{attribute 'qualified_only'}
VAR_GLOBAL
//######################## EL1809 ########################
	I_bTerm1_Var1 AT%I* : BOOL;		// Kitchen Light1
	I_bTerm1_Var2 AT%I* :  BOOL;	// Kitchen Light2
	I_bTerm1_Var3 AT%I* : BOOL;		// Kitchen Light3
	I_bTerm1_Var4 AT%I* : BOOL;		// Kitchen Blind Up
	I_bTerm1_Var5 AT%I* : BOOL;		// Kitchen Blind Down
	I_bTerm1_Var6 AT%I* : BOOL;
	I_bTerm1_Var7 AT%I* : BOOL;		// Corridor Light1
	I_bTerm1_Var8 AT%I* : BOOL;		// Corridor Light2
	I_bTerm1_Var9 AT%I* : BOOL;
	I_bTerm1_Var10 AT%I*:  BOOL;	// Livingroom Light1
	I_bTerm1_Var11 AT%I*:  BOOL;	// Livingroom Light2
	I_bTerm1_Var12 AT%I* : BOOL;	// Livingroom Light3
	I_bTerm1_Var13 AT%I* : BOOL;	// Livingroom Blind1 Up
	I_bTerm1_Var14 AT%I* : BOOL;	// Livingroom Blind1 Down
	I_bTerm1_Var15 AT%I* : BOOL;	// Livingroom Blind2 Up
	I_bTerm1_Var16 AT%I* : BOOL;	// Livingroom Blind2 Down
	
//######################## EL1809 ########################
	I_bTerm2_Var1 AT%I* : BOOL;		// Diningroom Light1
	I_bTerm2_Var2 AT%I* :  BOOL;	// Diningroom Light2
	I_bTerm2_Var3 AT%I* : BOOL;		// Diningroom Light3
	I_bTerm2_Var4 AT%I* : BOOL;		// Diningroom Blind1 Up
	I_bTerm2_Var5 AT%I* : BOOL;		// Diningroom Blind1 Down
	I_bTerm2_Var6 AT%I* : BOOL;		// Diningroom Blind2 Up
	I_bTerm2_Var7 AT%I* : BOOL;		// Diningroom Blind2 Down
	I_bTerm2_Var8 AT%I* : BOOL;
	I_bTerm2_Var9 AT%I* : BOOL;		// Bedroom Light1
	I_bTerm2_Var10 AT%I*:  BOOL;	// Bedroom Light2
	I_bTerm2_Var11 AT%I*:  BOOL;	// Bedroom Blind Up
	I_bTerm2_Var12 AT%I* : BOOL;	// Bedroom Blind Down
	I_bTerm2_Var13 AT%I* : BOOL;
	I_bTerm2_Var14 AT%I* : BOOL;	// Bath Light
	I_bTerm2_Var15 AT%I* : BOOL;	// Bath Blind Up
	I_bTerm2_Var16 AT%I* : BOOL;	// Bath Blind Down
	
//######################## EL2809 ########################
	Q_bTerm3_Var1 AT%Q* : BOOL;		// Kitchen Light1 ON
	Q_bTerm3_Var2 AT%Q* :  BOOL;	// Kitchen Light2 ON
	Q_bTerm3_Var3 AT%Q* : BOOL;		// Kitchen Light3 ON
	Q_bTerm3_Var4 AT%Q* : BOOL;		
	Q_bTerm3_Var5 AT%Q* : BOOL;		// Corridor Light1 ON
	Q_bTerm3_Var6 AT%Q* : BOOL;		// Corridor Light2 ON
	Q_bTerm3_Var7 AT%Q* : BOOL;
	Q_bTerm3_Var8 AT%Q* : BOOL;		// Livingroom Light1 ON
	Q_bTerm3_Var9 AT%Q* : BOOL;		// Livingroom Light2 ON
	Q_bTerm3_Var10 AT%Q*:  BOOL;	// Livingroom Light3 ON
	Q_bTerm3_Var11 AT%Q*:  BOOL;	
	Q_bTerm3_Var12 AT%Q* : BOOL;	// Diningroom Light1
	Q_bTerm3_Var13 AT%Q* : BOOL;	// Diningroom Light2
	Q_bTerm3_Var14 AT%Q* : BOOL;	// Diningroom Light3
	Q_bTerm3_Var15 AT%Q* : BOOL;
	Q_bTerm3_Var16 AT%Q* : BOOL;
	
//######################## EL2809 ########################
	Q_bTerm4_Var1 AT%Q* : BOOL;		// Bedroom Light1
	Q_bTerm4_Var2 AT%Q* :  BOOL;	// Bedroom Light2
	Q_bTerm4_Var3 AT%Q* : BOOL;
	Q_bTerm4_Var4 AT%Q* : BOOL;		// Bath Light
	Q_bTerm4_Var5 AT%Q* : BOOL;
	Q_bTerm4_Var6 AT%Q* : BOOL;
	Q_bTerm4_Var7 AT%Q* : BOOL;
	Q_bTerm4_Var8 AT%Q* : BOOL;
	Q_bTerm4_Var9 AT%Q* : BOOL;
	Q_bTerm4_Var10 AT%Q*:  BOOL;
	Q_bTerm4_Var11 AT%Q*:  BOOL;
	Q_bTerm4_Var12 AT%Q* : BOOL;
	Q_bTerm4_Var13 AT%Q* : BOOL;
	Q_bTerm4_Var14 AT%Q* : BOOL;
	Q_bTerm4_Var15 AT%Q* : BOOL;
	Q_bTerm4_Var16 AT%Q* : BOOL;
	
//######################## EL3204 ########################
	I_nTerm5_Var1 AT%I* : INT;			// Bath Temperature
	I_nTerm5_Var2 AT%I* : INT;			// Livingroom Temperature
	I_nTerm5_Var3 AT%I* : INT;			// Diningroom Temperature
	I_nTerm5_Var4 AT%I* : INT;			// Corridor Temperature
	
//######################## EL2722 ########################
	Q_bTerm6_Var1 AT%Q* : BOOL;			// Kitchen Blind Up
	Q_bTerm6_Var2 AT%Q* :  BOOL;		// Kitchen Blind Down
	
//######################## EL2722 ########################
	Q_bTerm7_Var1 AT%Q* : BOOL;			// Livingroom Blind1 Up
	Q_bTerm7_Var2 AT%Q* :  BOOL;		// Livingroom Blind1 Down
	
//######################## EL2722 ########################
	Q_bTerm8_Var1 AT%Q* : BOOL;			// Livingroom Blind2 Up
	Q_bTerm8_Var2 AT%Q* :  BOOL;		// Livingroom Blind2 Down
	
//######################## EL2722 ########################
	Q_bTerm9_Var1 AT%Q* : BOOL;			// Diningroom Blind1 Up
	Q_bTerm9_Var2 AT%Q* :  BOOL;		// Diningroom Blind1 Down
	
//######################## EL2722 ########################
	Q_bTerm10_Var1 AT%Q* : BOOL;		// Diningroom Blind2 Up
	Q_bTerm10_Var2 AT%Q* :  BOOL;		// Diningroom Blind2 Down
	
//######################## EL2722 ########################
	Q_bTerm11_Var1 AT%Q* : BOOL;		// Bedroom Blind Up
	Q_bTerm11_Var2 AT%Q* :  BOOL;		// Bedroom Blind Down
	
//######################## EL2722 ########################
	Q_bTerm12_Var1 AT%Q* : BOOL;		// Bath Blind Up
	Q_bTerm12_Var2 AT%Q* :  BOOL;		// Bath Blind Down
	
//######################## EL3403 ########################
	I_nTerm13_Voltage1 AT%I* : DINT;
	I_nTerm13_Voltage2 AT%I* : DINT;
	I_nTerm13_Voltage3 AT%I* : DINT;
	I_nTerm13_Current1 AT%I* : DINT;
	I_nTerm13_Current2 AT%I* : DINT;
	I_nTerm13_Current3 AT%I* : DINT;
	I_nTerm13_Power1 AT%I* : DINT;
	I_nTerm13_Power2 AT%I* : DINT;
	I_nTerm13_Power3 AT%I* : DINT;
END_VAR
